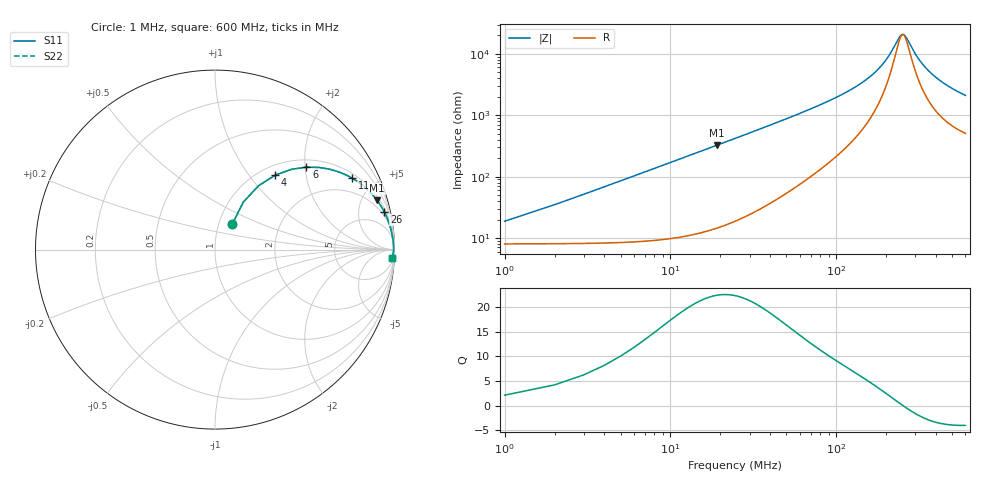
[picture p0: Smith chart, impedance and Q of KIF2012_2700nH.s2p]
!version-2
!date-12.2020
!Series
# MHz S RI R 50
!Freq ReS11 ImS11 ReS21 ImS21 ReS12 ImS12 ReS22 ImS22
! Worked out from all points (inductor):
!   600 points, 1 MHz to 600 MHz, reference 50 ohm
!   read as one part in series: L = 2.7 uH near 4 MHz
!   highest Q = 22.3 at 19 MHz (marker M1), where L = 2.71 uH
!   self-resonance near 252.2 MHz
!   S11 on the Smith chart (normalised r, x): 1 MHz: 1.16, +0.34; 4 MHz: 1.17, +1.36; 6 MHz: 1.17, +2.03; 11 MHz: 1.20, +3.73; 26 MHz: 1.40, +8.89; 600 MHz: 11, -41
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1  0.0963 0.1418  0.9037 -0.1418  0.9037 -0.1418  0.0963 0.1418
4  0.3366 0.4155  0.6634 -0.4155  0.6634 -0.4155  0.3366 0.4155
5  0.4276 0.4475  0.5724 -0.4475  0.5724 -0.4475  0.4276 0.4475
6  0.5096 0.4593  0.4904 -0.4593  0.4904 -0.4593  0.5096 0.4593
8  0.6401 0.4475  0.3599 -0.4475  0.3599 -0.4475  0.6401 0.4475
11  0.7656 0.3973  0.2344 -0.3973  0.2344 -0.3973  0.7656 0.3973
14  0.8384 0.3447  0.1616 -0.3447  0.1616 -0.3447  0.8384 0.3447
19  0.9028 0.2748  0.0972 -0.2748  0.0972 -0.2748  0.9028 0.2748
26  0.9433 0.2098  0.0567 -0.2098  0.0567 -0.2098  0.9433 0.2098
38  0.9701 0.1464  0.0299 -0.1464  0.0299 -0.1464  0.9701 0.1464
54  0.9826 0.1024  0.0174 -0.1024  0.0174 -0.1024  0.9826 0.1024
101  0.992 0.0494  0.00798 -0.0494  0.00798 -0.0494  0.992 0.0494
165  0.9948 0.021  0.00524 -0.021  0.00524 -0.021  0.9948 0.021
201  0.9952 0.0111  0.00479 -0.0111  0.00479 -0.0111  0.9952 0.0111
237  0.9953 0.00303  0.00474 -0.00303  0.00474 -0.00303  0.9953 0.00303
250  0.9952 0.000421  0.00479 -0.000421  0.00479 -0.000421  0.9952 0.000421
263  0.9951 -0.00205  0.00489 0.00205  0.00489 0.00205  0.9951 -0.00205
301  0.9947 -0.00868  0.00532 0.00868  0.00532 0.00868  0.9947 -0.00868
344  0.9939 -0.0153  0.00607 0.0153  0.00607 0.0153  0.9939 -0.0153
401  0.9926 -0.0232  0.00736 0.0232  0.00736 0.0232  0.9926 -0.0232
501  0.9898 -0.035  0.0102 0.035  0.0102 0.035  0.9898 -0.035
600  0.9866 -0.045  0.0134 0.045  0.0134 0.045  0.9866 -0.045
